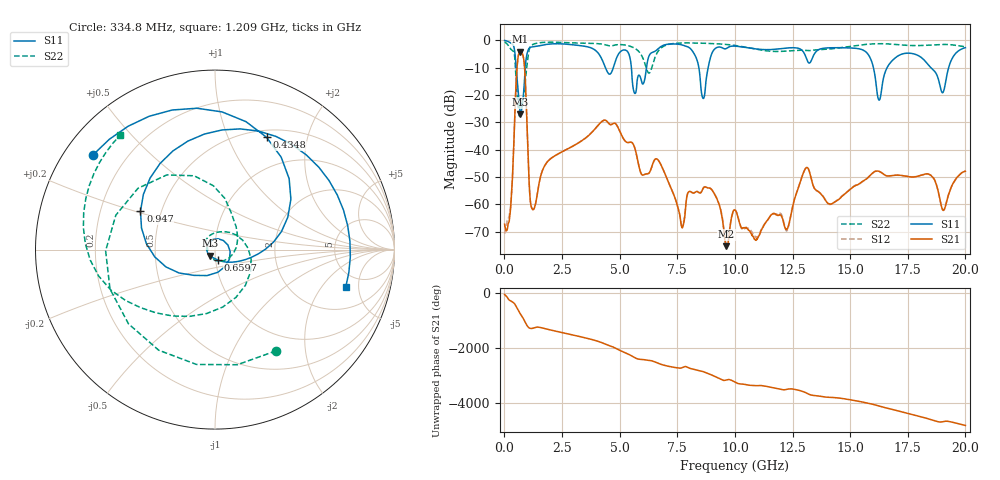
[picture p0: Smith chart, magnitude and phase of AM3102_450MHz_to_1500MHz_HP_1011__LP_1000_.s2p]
!Agilent Technologies,E8364B,MY43040894,A.07.50.67
!Agilent E8364B: A.07.50.67
!Date: Thursday, January 11, 2018 06:25:03
!Correction: S11(Full 2 Port(1,2))
!S21(Full 2 Port(1,2))
!S12(Full 2 Port(1,2))
!S22(Full 2 Port(1,2))
!S2P File: Measurements: S11, S21, S12, S22:
# Hz S  dB  R 50
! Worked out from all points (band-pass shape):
!   1601 points, 10 MHz to 20 GHz, reference 50 ohm
!   highest |S21| = -4.15 dB at 697.2 MHz (marker M1); lowest = -75.4 dB at 9.63 GHz (marker M2)
!   |S21| within 3 dB of the highest: 579.6 MHz to 844.4 MHz (264.9 MHz wide, 37.2 % of centre)
!   lowest |S11| = -27.0 dB at 697.2 MHz (marker M3), VSWR 1.09, Z = 47 - j3.15 ohm
!   |S11| at or under -10 dB: 5.51 GHz to 6.165 GHz (654.7 MHz wide, 11.2 % of centre); 16.01 GHz to 16.6 GHz (593 MHz wide, 3.64 % of centre); 18.5 GHz to 19.27 GHz (772.1 MHz wide, 4.09 % of centre)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
!   |S22| runs from -28.2 to -0.6 dB; largest |S21 - S12| = 0.001
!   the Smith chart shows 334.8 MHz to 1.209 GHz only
!   S11 on the Smith chart (normalised r, x): 334.8 MHz: 0.08, +0.34; 434.8 MHz: 0.58, +1.39; 659.7 MHz: 1.02, -0.12; 947 MHz: 0.38, +0.21; 1.209 GHz: 3.60, -3.56
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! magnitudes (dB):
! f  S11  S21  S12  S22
! 10 MHz  0.0  -67.3  -70.8  -0.6
! 334.8 MHz  -1.3  -52.9  -52.5  -3.6
! 434.8 MHz  -3.2  -31.6  -31.5  -5.2
! 659.7 MHz  -24.5  -4.3  -4.3  -28.2
! 697.2 MHz  -27.0  -4.1  -4.1  -27.2
! 947 MHz  -6.6  -22.8  -22.8  -11.7
! 1.209 GHz  -2.4  -61.8  -61.6  -1.6
! 3.346 GHz  -2.0  -36.8  -36.8  -1.0
! 5.295 GHz  -3.7  -37.3  -37.3  -1.8
! 5.657 GHz  -19.4  -39.4  -39.4  -2.9
! 6.682 GHz  -3.0  -43.9  -44.0  -3.9
! 7.719 GHz  -1.7  -68.7  -67.7  -1.0
! 8.618 GHz  -21.2  -54.3  -54.2  -1.1
! 9.63 GHz  -3.0  -75.4  -74.7  -1.5
! 10.01 GHz  -2.1  -62.2  -62.0  -1.9
! 12.27 GHz  -2.8  -69.1  -69.6  -3.9
! 13.34 GHz  -6.9  -51.6  -51.5  -3.7
! 15.59 GHz  -3.7  -51.4  -51.5  -1.6
! 16.25 GHz  -21.9  -48.0  -48.0  -1.2
! 16.68 GHz  -9.0  -49.7  -49.6  -1.3
! 19.01 GHz  -19.2  -62.0  -62.1  -1.5
! 20 GHz  -2.7  -47.9  -47.7  -2.3
